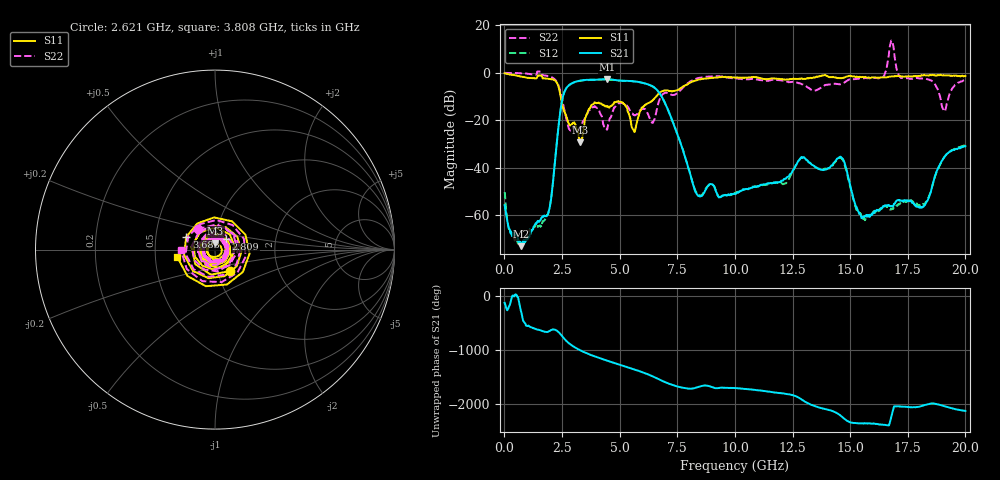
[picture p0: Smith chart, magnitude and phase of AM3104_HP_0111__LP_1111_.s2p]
!Created with skrf (http://scikit-rf.org).
# Hz S RI R 50.0
!freq ReS11 ImS11 ReS21 ImS21 ReS12 ImS12 ReS22 ImS22
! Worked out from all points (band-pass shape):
!   1601 points, 10 MHz to 20 GHz, reference 50 ohm
!   highest |S21| = -2.71 dB at 4.458 GHz (marker M1); lowest = -72.9 dB at 734.6 MHz (marker M2)
!   |S21| within 3 dB of the highest: 2.751 GHz to 6.438 GHz (3.687 GHz wide, 80.3 % of centre)
!   lowest |S11| = -29.2 dB at 3.283 GHz (marker M3), VSWR 1.07, Z = 50.1 + j3.46 ohm
!   |S11| at or under -10 dB: 2.441 GHz to 6.584 GHz (4.143 GHz wide, 91.8 % of centre)
!   |S22| runs from -24.3 to 13.6 dB; largest |S21 - S12| = 0.082
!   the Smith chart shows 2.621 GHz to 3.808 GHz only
!   S11 on the Smith chart (normalised r, x): 2.621 GHz: 1.14, -0.28; 2.809 GHz: 1.12, +0.13; 3.683 GHz: 0.72, +0.10; 3.808 GHz: 0.65, -0.06
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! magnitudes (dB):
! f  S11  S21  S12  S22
! 10 MHz  -0.2  -55.7  -50.2  0.0
! 734.6 MHz  -1.6  -72.9  -72.6  -0.3
! 1.922 GHz  -2.5  -58.2  -58.5  -1.4
! 2.621 GHz  -16.7  -7.7  -7.6  -16.5
! 2.809 GHz  -21.6  -5.2  -5.2  -23.7
! 3.283 GHz  -29.2  -3.3  -3.4  -23.2
! 3.346 GHz  -27.8  -3.2  -3.3  -22.5
! 3.683 GHz  -15.1  -2.9  -3.0  -15.6
! 3.808 GHz  -13.4  -2.9  -2.9  -14.5
! 4.458 GHz  -14.1  -2.7  -2.7  -23.9
! 4.958 GHz  -12.0  -3.2  -3.3  -12.7
! 5.62 GHz  -24.4  -3.6  -3.6  -17.7
! 6.682 GHz  -8.9  -7.9  -7.9  -12.6
! 8.368 GHz  -3.1  -51.3  -50.8  -2.3
! 10.01 GHz  -2.0  -50.9  -50.6  -2.4
! 13.34 GHz  -2.2  -38.6  -38.6  -7.3
! 14.64 GHz  -2.2  -35.8  -36.2  -4.7
! 15.53 GHz  -1.7  -60.8  -61.4  -2.3
! 16.68 GHz  -1.7  -55.8  -57.0  7.3
! 18.18 GHz  -1.0  -56.3  -55.3  -2.4
! 19.06 GHz  -1.1  -35.8  -35.7  -15.7
! 20 GHz  -1.4  -30.9  -30.3  -3.0
